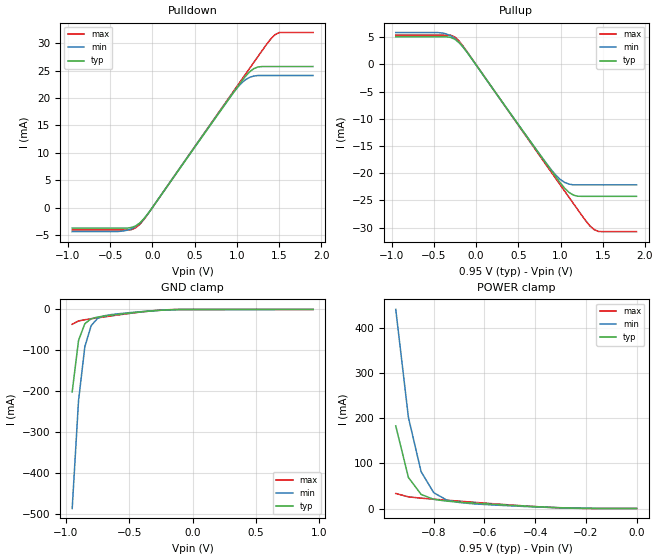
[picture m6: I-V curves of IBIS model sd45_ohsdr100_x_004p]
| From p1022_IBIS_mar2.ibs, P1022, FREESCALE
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[Model]   sd45_ohsdr100_x_004p
Model_type 3-state
Enable Active-High
Polarity Non-Inverting
|   TYP   MIN   MAX
C_comp   1.60pF   1.60pF   1.67pF
[Model Spec]
Vmeas   0.475   0.425   0.605
[Voltage Range]   0.95   0.85   1.21
[Temperature Range] 65   125   -40
[Driver Schedule]
| Model_Name  Rise_on_dly   Rise_off_dly   Fall_on_dly   Fall_off_dly
sd45_ohsdr100_x_00   0ps   NA   0ps   NA
sd45_ohsdr100_x_04   400ps   NA   400ps   NA
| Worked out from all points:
|   slope of the pulldown table from 0 to 0.142 V, typ, clamps not added: 45.5 ohm
|   slope of the pullup table from 0 to 0.142 V, typ, clamps not added: 45.4 ohm
|   GND clamp passes 1 mA (typ) near -0.19 V on its own axis
|   POWER clamp passes 1 mA (typ) near -0.25 V on its own axis
[Pullup]
|   Vout(V)   TYP   WCS   BCS
-950mV    5.093mA    5.874mA    5.386mA
-400mV    5.093mA    5.787mA    5.386mA
-250mV    4.634mA    4.784mA    5.037mA
-100mV    2.128mA    2.126mA    2.211mA
750mV     -16.46mA   -16.43mA   -16.69mA
900mV     -19.71mA   -19.54mA   -20.01mA
1V        -21.82mA   -21.19mA   -22.22mA
1.15V     -24mA      -22.13mA   -25.52mA
1.3V      -24.25mA   -22.13mA   -28.77mA
1.4V      -24.25mA   -22.13mA   -30.39mA
1.45V     -24.25mA   -22.13mA   -30.72mA
1.9V      -24.25mA   -22.13mA   -30.75mA
[Pulldown]
|   Vout(V)   TYP   WCS   BCS
-950mV    -3.758mA   -4.406mA   -4.109mA
-400mV    -3.758mA   -4.371mA   -4.109mA
-200mV    -3.361mA   -3.47mA    -3.717mA
-50mV     -1.064mA   -1.064mA   -1.095mA
900mV     19.7mA     19.76mA    19.92mA
1V        21.87mA    21.8mA     22.11mA
1.1V      23.93mA    23.32mA    24.31mA
1.2V      25.36mA    24.01mA    26.5mA
1.25V     25.67mA    24.1mA     27.6mA
1.45V     25.74mA    24.1mA     31.55mA
1.5V      25.74mA    24.1mA     31.94mA
1.9V      25.74mA    24.1mA     31.94mA
[GND Clamp]
|   Vout(V)   TYP   WCS   BCS
-950mV    -201.6mA   -486.5mA   -36.16mA
-900mV    -75.75mA   -222.9mA   -28.05mA
-850mV    -34.66mA   -90.59mA   -25.11mA
-800mV    -22.71mA   -39.37mA   -22.78mA
-750mV    -18.57mA   -21.91mA   -20.52mA
-700mV    -16.25mA   -15.71mA   -18.29mA
-650mV    -14.32mA   -12.88mA   -16.07mA
-400mV    -5.858mA   -5.175mA   -5.911mA
-200mV    -1.108mA   -1.072mA   -756.7uA
950mV     70.01uA    122.9uA    16.34uA
[POWER Clamp]
|   Vout(V)   TYP   WCS   BCS
-950mV    183.5mA    442.2mA    33.42mA
-900mV    68.86mA    202.2mA    25.88mA
-850mV    31.34mA    81.75mA    23.04mA
-800mV    20.35mA    35.06mA    20.76mA
-750mV    16.46mA    19.08mA    18.55mA
-700mV    14.22mA    13.35mA    16.36mA
-650mV    12.35mA    10.71mA    14.18mA
-300mV    1.805mA    1.56mA     1.409mA
0V        0A         0A         0A
[Ramp]
R_load=50.00
dV/dt_r  2.9887e-01/6.4040e-11  2.6861e-01/6.5155e-11  3.8214e-01/6.5744e-11
dV/dt_f  2.9887e-01/6.6355e-11  2.6861e-01/6.7761e-11  3.8218e-01/6.7348e-11
